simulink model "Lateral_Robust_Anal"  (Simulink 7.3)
settings: Solver=ode45  StartTime=0.0  StopTime=44  RelTol=1e-3
InitFcn:
  | init
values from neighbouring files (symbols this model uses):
  calfa = cos(alfa0*d2r)    [init.m]
  d2r = pi/180    (= 0.0174532925199)    [init.m]    (also in robust.m)
  ge = 32.174    [init.m]
  r2d = 180/pi    (= 57.2957795131)    [init.m]    (also in robust.m)
  salfa = sin(alfa0*d2r)    [init.m]
  Thet0 = 27.69    [init.m]
  V0 = 24675.1    [init.m]
undefined symbols (not defined in the file or in its folder): Alu, Blu, Clu, Dlu, Kmix, Kpr

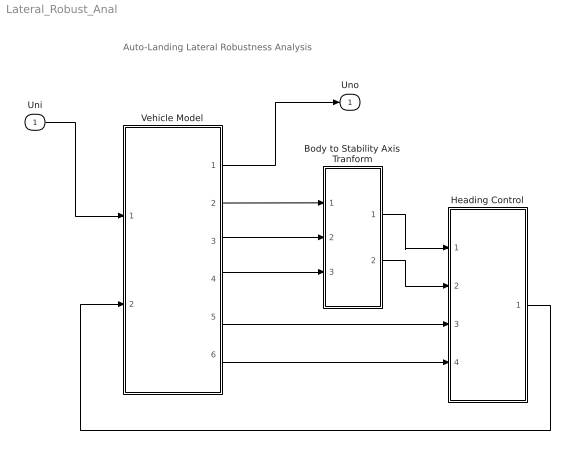
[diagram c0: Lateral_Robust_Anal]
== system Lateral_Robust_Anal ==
  note: Auto-Landing Lateral Robustness Analysis
  Uni : Inport  OutDataType=sfix(16)  OutScaling=2^0
  Body to Stability Axis Tranform : Subsystem
  Heading Control : Subsystem
  Vehicle Model : Subsystem
  Uno : Outport  OutDataType=sfix(16)  OutScaling=2^0
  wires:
  Vehicle Model/1(Uno) -> Uno/1
  Uni/1 -> Vehicle Model/1(Uni)
  Vehicle Model/2(phi) -> Body to Stability Axis Tranform/1(phi)
  Vehicle Model/3(p) -> Body to Stability Axis Tranform/2(p_b)
  Vehicle Model/4(r) -> Body to Stability Axis Tranform/3(r_b)
  Vehicle Model/6(Vcr) -> Heading Control/4(Vcr)
  Vehicle Model/5(Ny) -> Heading Control/3(Ny)
  Body to Stability Axis Tranform/2(r_s) -> Heading Control/2(rs)
  Body to Stability Axis Tranform/1(p_s) -> Heading Control/1(ps)
  Heading Control/1((dP,dR)) -> Vehicle Model/2("(dP, dR)")

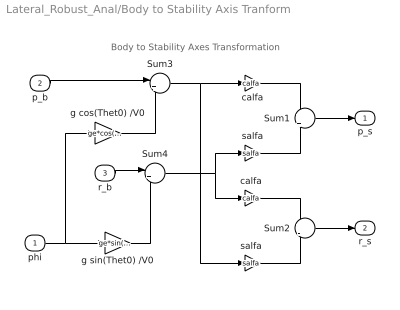
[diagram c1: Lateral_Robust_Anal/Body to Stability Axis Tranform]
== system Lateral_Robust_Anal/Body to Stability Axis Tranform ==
  note: Body to Stability Axes Transformation
  phi : Inport  OutDataType=sfix(16)  OutScaling=2^0
  p_b : Inport  Port=2  OutDataType=sfix(16)  OutScaling=2^0
  r_b : Inport  Port=3  OutDataType=sfix(16)  OutScaling=2^0
  Sum1 : Sum  Inputs=+|+  OutDataType=sfix(16)  OutScaling=2^0
  Sum2 : Sum  Inputs=+|-  OutDataType=sfix(16)  OutScaling=2^0
  Sum3 : Sum  Inputs=|++  OutDataType=sfix(16)  OutScaling=2^0
  Sum4 : Sum  Inputs=|+-  OutDataType=sfix(16)  OutScaling=2^0
  calfa : Gain  Gain=calfa  ParameterDataType=sfix(16)  ParameterScaling=2^0  OutDataType=sfix(16)  OutScaling=2^0
  "calfa " : Gain  Gain=calfa  ParameterDataType=sfix(16)  ParameterScaling=2^0  OutDataType=sfix(16)  OutScaling=2^0
  g cos(Thet0) /V0 : Gain  Gain=ge*cos(Thet0*d2r)/V0  ParameterDataType=sfix(16)  ParameterScaling=2^0  OutDataType=sfix(16)  OutScaling=2^0
  g sin(Thet0) /V0 : Gain  Gain=ge*sin(Thet0*d2r)/V0  ParameterDataType=sfix(16)  ParameterScaling=2^0  OutDataType=sfix(16)  OutScaling=2^0
  salfa : Gain  Gain=salfa  ParameterDataType=sfix(16)  ParameterScaling=2^0  OutDataType=sfix(16)  OutScaling=2^0
  "salfa " : Gain  Gain=salfa  ParameterDataType=sfix(16)  ParameterScaling=2^0  OutDataType=sfix(16)  OutScaling=2^0
  p_s : Outport  OutDataType=sfix(16)  OutScaling=2^0
  r_s : Outport  Port=2  OutDataType=sfix(16)  OutScaling=2^0
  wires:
  "salfa "/1 -> Sum2/2
  "calfa "/1 -> Sum2/1
  salfa/1 -> Sum1/2
  calfa/1 -> Sum1/1
  Sum3/1 -> calfa/1, "salfa "/1
  Sum4/1 -> salfa/1, "calfa "/1
  phi/1 -> g sin(Thet0) /V0/1, g cos(Thet0) /V0/1
  g sin(Thet0) /V0/1 -> Sum4/2
  g cos(Thet0) /V0/1 -> Sum3/2
  r_b/1 -> Sum4/1
  p_b/1 -> Sum3/1
  Sum2/1 -> r_s/1
  Sum1/1 -> p_s/1

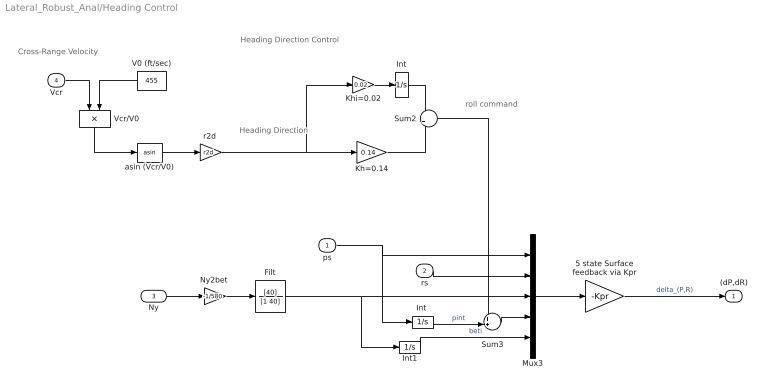
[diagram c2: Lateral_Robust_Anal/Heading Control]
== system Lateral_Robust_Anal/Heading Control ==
  note: Cross-Range Velocity
  note: Heading Direction
  note: roll command
  note: Heading Direction Control
  ps : Inport  OutDataType=sfix(16)  OutScaling=2^0
  rs : Inport  Port=2  OutDataType=sfix(16)  OutScaling=2^0
  Ny : Inport  Port=3
  Vcr : Inport  Port=4  OutDataType=sfix(16)  OutScaling=2^0
  5 state Surface feedback via Kpr : Gain  Gain=-Kpr  Multiplication=Matrix(K*u)  ParameterDataType=sfix(16)  ParameterScaling=2^0  OutDataType=sfix(16)  OutScaling=2^0
  Filt : TransferFcn  Numerator=[40]  Denominator=[1 40]
  Int : Integrator
  "Int " : Integrator
  Int1 : Integrator
  Kh=0.14 : Gain  Gain=0.14  ParameterDataType=sfix(16)  ParameterScaling=2^0  OutDataType=sfix(16)  OutScaling=2^0
  Khi=0.02 : Gain  Gain=0.02  ParameterDataType=sfix(16)  ParameterScaling=2^0  OutDataType=sfix(16)  OutScaling=2^0
  Mux3 : Mux  Inputs=5
  "Ny2bet " : Gain  Gain=-1/580  ParameterDataType=sfix(16)  ParameterScaling=2^0  OutDataType=sfix(16)  OutScaling=2^0
  Sum2 : Sum  OutDataType=sfix(16)  OutScaling=2^0
  Sum3 : Sum  Inputs=++|  OutDataType=sfix(16)  OutScaling=2^0
  V0 (ft/sec) : Constant  Value=455  OutDataType=sfix(16)  OutScaling=2^0
  Vcr/V0 : Product  Inputs=*/  OutDataType=sfix(16)  OutScaling=2^0
  asin (Vcr/V0) : Trigonometry  Operator=asin
  "r2d " : Gain  Gain=r2d  ParameterDataType=sfix(16)  ParameterScaling=2^0  OutDataType=sfix(16)  OutScaling=2^0
  (dP,dR) : Outport  OutDataType=sfix(16)  OutScaling=2^0
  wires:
  Filt/1 -> Mux3/3, Int1/1
  Ny/1 -> "Ny2bet "/1
  "Ny2bet "/1 -> Filt/1
  "Int "/1 -> Sum3/2  "pint"
  Sum3/1 -> Mux3/4
  Int1/1 -> Mux3/5  "beti"
  ps/1 -> Mux3/1, "Int "/1
  rs/1 -> Mux3/2
  5 state Surface feedback via Kpr/1 -> (dP,dR)/1  "delta_(P,R)"
  Mux3/1 -> 5 state Surface feedback via Kpr/1
  V0 (ft/sec)/1 -> Vcr/V0/2
  asin (Vcr/V0)/1 -> "r2d "/1
  Vcr/V0/1 -> asin (Vcr/V0)/1
  "r2d "/1 -> Khi=0.02/1, Kh=0.14/1
  Khi=0.02/1 -> Int/1
  Kh=0.14/1 -> Sum2/2
  Int/1 -> Sum2/1
  Vcr/1 -> Vcr/V0/1
  Sum2/1 -> Sum3/1

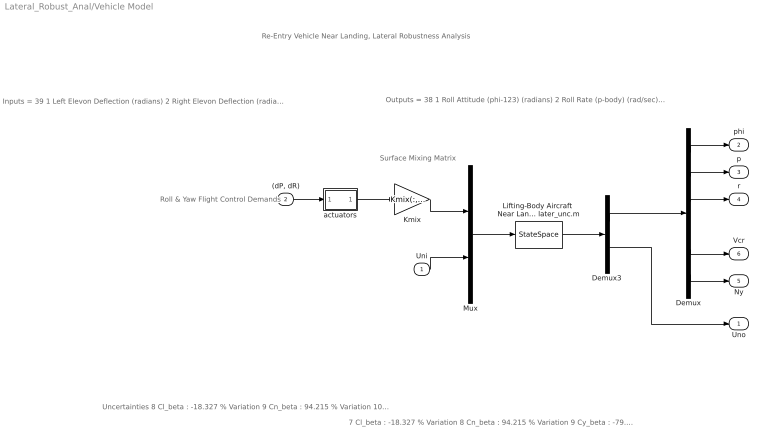
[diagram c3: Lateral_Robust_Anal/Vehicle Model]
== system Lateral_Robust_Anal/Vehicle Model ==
  note: Re-Entry Vehicle Near Landing, Lateral Robustness Analysis
  note: Surface Mixing Matrix
  note: Roll & Yaw Flight Control Demands
  note: Inputs = 39 1 Left Elevon Deflection (radians) 2 Right Elevon Deflection (radians) 3 Vertical Rudder Deflection (radians) 4 Upper Left Body-Flap Deflection (radians) 5 Upper Right Body-Flap Deflection (radians) 6 Lower Left Body-Flap Deflection (radians) 7 Lower Right Body-Flap Deflection (radians)
  note: Uncertainties 8 Cl_beta : -18.327 % Variation 9 Cn_beta : 94.215 % Variation 10 Cy_beta : -79.319 % Variation 11 Cn_p : 33.213 % Variation 12 Cn_r : -10.061 % Variation 13 Cl_p : -16.577 % Variation 14 Cl_r : 7.489 % Variation 15 I_xx : 4.630 % Variation 16 I_zz : 4.032 % Variation 17 Xcg locat: -2.934 % Variation 18 Ycg locat: 0.5 Additive Variat. 19 Cy_surf 1: 119.180 % Variation 20 Cl_surf 1: 42.758 % Variation 21 Cn_surf 1: -75.811 % Variation 22 Cy_surf 2: -119.180 % Variation 23 Cl_surf 2: -42.758 % Variation 24 Cn_surf 2: 75.811 % Variation 25 Cy_surf 3: 45.974 % Variation 26 Cl_surf 3: 192.469 % Variation 27 Cn_surf 3: -26.230 % Variation 28 Cy_surf 4: -79.923 % Variation 29 Cl_surf 4: 44.556 % Variation 30 Cn_surf 4: 372.283 % Variation 31 Cy_surf 5: 79.923 % Variation 32 Cl_surf 5: -44.556 % Variation 33 Cn_surf 5: -372.283 % Variation 34 Cy_surf 6: 33.642 % Variation 35 Cl_surf 6: 32.372 % Variation 36 Cn_surf 6: -51.630 % Variation 37 Cy_surf 7: -33.642 % Variation 38 Cl_surf 7: -32.372 % Variation 39 Cn_surf 7: 51.630 % Variation
  note: Outputs = 38 1 Roll Attitude (phi-123) (radians) 2 Roll Rate (p-body) (rad/sec) 3 Yaw Rate (r-body) (rad/sec) 4 Angle of sideslip, beta, (radian) 5 Cross Range Velocity (Vcr) (ft/sec) 6 Accelerom #2, (along Y), (ft/sec^2)
  note: 7 Cl_beta : -18.327 % Variation 8 Cn_beta : 94.215 % Variation 9 Cy_beta : -79.319 % Variation 10 Cn_p : 33.213 % Variation 11 Cn_r : -10.061 % Variation 12 Cl_p : -16.577 % Variation 13 Cl_r : 7.489 % Variation 14 I_xx : 4.630 % Variation 15 I_zz : 4.032 % Variation 16 Xcg locat: -2.934 % Variation 17 Ycg locat: 0.5 Additive Variation 18 Cy_surf 1: 119.180 % Variation 19 Cl_surf 1: 42.758 % Variation 20 Cn_surf 1: -75.811 % Variation 21 Cy_surf 2: -119.180 % Variation 22 Cl_surf 2: -42.758 % Variation 23 Cn_surf 2: 75.811 % Variation 24 Cy_surf 3: 45.974 % Variation 25 Cl_surf 3: 192.469 % Variation 26 Cn_surf 3: -26.230 % Variation 27 Cy_surf 4: -79.923 % Variation 28 Cl_surf 4: 44.556 % Variation 29 Cn_surf 4: 372.283 % Variation 30 Cy_surf 5: 79.923 % Variation 31 Cl_surf 5: -44.556 % Variation 32 Cn_surf 5: -372.283 % Variation 33 Cy_surf 6: 33.642 % Variation 34 Cl_surf 6: 32.372 % Variation 35 Cn_surf 6: -51.630 % Variation 36 Cy_surf 7: -33.642 % Variation 37 Cl_surf 7: -32.372 % Variation 38 Cn_surf 7: 51.630 % Variation
  Uni : Inport  OutDataType=sfix(16)  OutScaling=2^0
  "(dP, dR)" : Inport  Port=2  OutDataType=sfix(16)  OutScaling=2^0
  Demux : Demux  Outputs=6
  Demux3 : Demux  Outputs=[6, 32]
  Kmix : Gain  Gain=Kmix(:,[1,3])  Multiplication=Matrix(K*u)  ParameterDataType=sfix(16)  ParameterScaling=2^0  OutDataType=sfix(16)  OutScaling=2^0
  "Lifting-Body Aircraft  Near Landing,  Lateral Robust Analysis  (32 Uncs) from file later_unc.m" : StateSpace  A=Alu  B=Blu  C=Clu  D=Dlu
  Mux : Mux  Inputs=[7, 32]
  actuators : Subsystem
  Uno : Outport  OutDataType=sfix(16)  OutScaling=2^0
  phi : Outport  Port=2  OutDataType=sfix(16)  OutScaling=2^0
  p : Outport  Port=3  OutDataType=sfix(16)  OutScaling=2^0
  r : Outport  Port=4  OutDataType=sfix(16)  OutScaling=2^0
  Ny : Outport  Port=5  OutDataType=sfix(16)  OutScaling=2^0
  Vcr : Outport  Port=6  OutDataType=sfix(16)  OutScaling=2^0
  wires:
  Mux/1 -> "Lifting-Body Aircraft  Near Landing,  Lateral Robust Analysis  (32 Uncs) from file later_unc.m"/1
  Kmix/1 -> Mux/1
  "(dP, dR)"/1 -> actuators/1(In)
  Uni/1 -> Mux/2
  "Lifting-Body Aircraft  Near Landing,  Lateral Robust Analysis  (32 Uncs) from file later_unc.m"/1 -> Demux3/1
  Demux3/1 -> Demux/1
  Demux3/2 -> Uno/1
  actuators/1(out) -> Kmix/1
  Demux/1 -> phi/1
  Demux/2 -> p/1
  Demux/3 -> r/1
  Demux/6 -> Ny/1
  Demux/5 -> Vcr/1

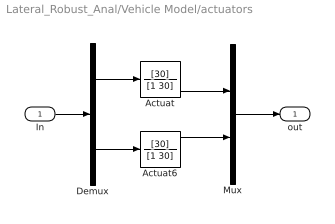
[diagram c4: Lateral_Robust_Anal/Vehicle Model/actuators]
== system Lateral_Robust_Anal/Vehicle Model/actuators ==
  In : Inport
  Actuat : TransferFcn  Numerator=[30]  Denominator=[1 30]
  Actuat6 : TransferFcn  Numerator=[30]  Denominator=[1 30]
  Demux : Demux  Outputs=2
  Mux : Mux  Inputs=2
  out : Outport
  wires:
  Actuat6/1 -> Mux/2
  Actuat/1 -> Mux/1
  Demux/2 -> Actuat6/1
  Demux/1 -> Actuat/1
  Mux/1 -> out/1
  In/1 -> Demux/1
